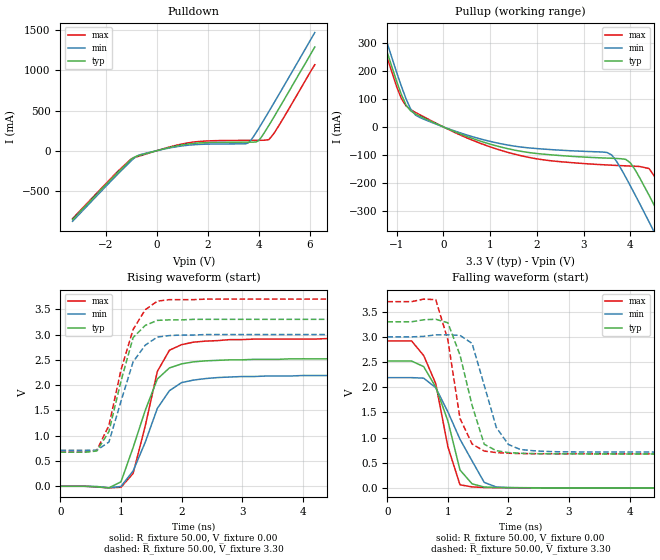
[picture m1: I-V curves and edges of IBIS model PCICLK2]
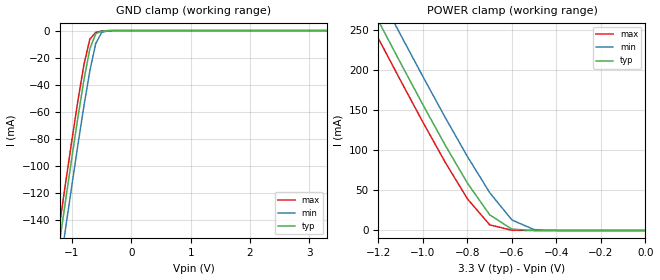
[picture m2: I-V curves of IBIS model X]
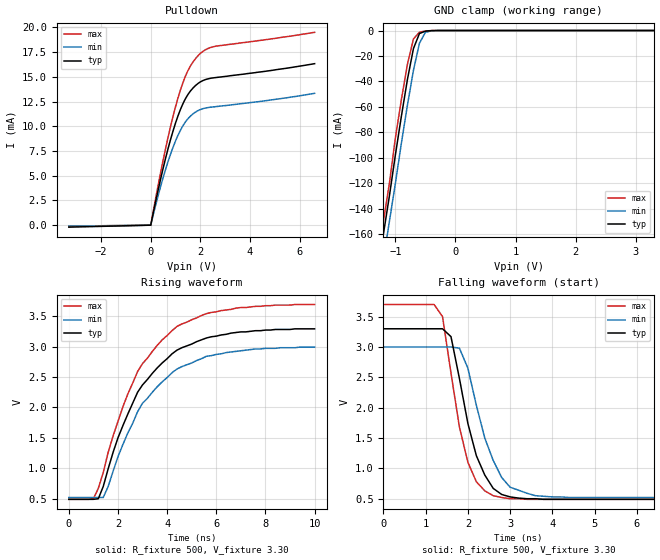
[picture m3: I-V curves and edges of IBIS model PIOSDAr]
|   * 9250-28.ibs * IBIS 2.1 Model for ICS9250-28
| Rev History
| Rev No.   Description
| 1.0   Initial release with Updated Parasitic Parameters
[IBIS Ver]   2.1
[Comment char]  |_char
[File name]   9250-28.ibs
[Date]   Aug 15, 2002
[File Rev]   1.1
[Source]   Originated at Integrated Circuit Systems, Inc.
[Disclaimer]
(C) Copyright Integrated Circuit Systems, Inc. 1997
   All rights reserved
ICS hereby grants the user of this IBIS model a non-exclusive,
nontransferable license to use this IBIS model under the following terms.
Before using this IBIS model, the user should read this license.
If the user does not accept these terms,  the IBIS model should be
returned to ICS within 30 days.
   The user is granted this license only to use the IBIS model and
is not granted rights to sell, load, rent, lease or license the IBIS
model in whole or in part, or in modified form to anyone other than
user. User may modify the IBIS model to suit its specific
applications but rights to derivative works and such modifications
shall belong to ICS.
   This IBIS model is provided on an "AS IS" basis and ICS makes
absolutely no warranty with respect to the information contained
herein. ICS DISCLAIMS AND CUSTOMER WAIVES ALL WARRANTIES, EXPRESS
OR IMPLIED, INCLUDING WARRANTIES OF MERCHANTABILITY OR FITNESS FOR
A PARTICULAR PURPOSE. The entire risk as to quality and performance
is with the Customer. ACCORDINGLY, IN NO EVENT SHALL THE COMPANY BE
LIABLE FOR ANY DAMAGES, WHETHER IN CONTRACT OR TORT,INCLUDING ANY
LOST PROFITS OR OTHER INCIDENTAL, CONSEQUENTIAL, EXEMPLARY, OR
PUNITIVE DAMAGES ARISING OUT OF THE USE OR APPLICATION OF THE IBIS
model provided in this package. Further, ICS reserves the right to
make changes without notice to any product herein to improve
reliability, function, or design. ICS does not convey any license
under patent rights or any other intellectual property rights,
including those of third parties.
   ICS is not obligated to provide maintenance or support
for the licensed IBIS model.
|   COMPONENT: ICS9250-28
[Component]   ICS9250-28
[Manufacturer]  ICS
[Package]
| variable   typ   min   max
R_pkg   81.1m   62.2m   100.0m
L_pkg   6.7nH   4.9nH   8.5nH
C_pkg   0.53pF  0.21pF  0.85pF
[Pin]   signal_name   model_name   R_pin   L_pin   C_pin
1   IOAPIC   IOAPIC
2   VDDL   POWER
3   GNDL   GND
4   FS2/REF0   PIO17
5   VDD   POWER
6   X1   X
7   X2   X
8   GND   GND
9   VDD   POWER
10   3V66-0   3V661
11   3V66-1   3V661
12   3V66-2   3V661
13   GND   GND
14   VDD   POWER
15   PCICLK0   PCICLK2
16   PCICLK1   PCICLK2
17   GND   GND
18   FS0   FS
19   GND   GND
20   VDD   POWER
21   PD#   PD
22   SCLK   SCLK
23   SDATA   PIOSDAr
24   GND   GND
25   VDD   POWER
26   48MHz_0   48MH
27   48MHz_1   48MHz2
28   FS1   FS
29   SDRAM12   SDRAM5
30   GND   GND
31   VDD   POWER
32   SDRAM11   SDRAM5
33   SDRAM10   SDRAM5
34   GND   GND
35   VDD   POWER
36   SDRAM9   SDRAM5
37   SDRAM8   SDRAM5
38   SDRAM7   SDRAM5
39   GND   GND
40   VDD   POWER
41   SDRAM6   SDRAM5
42   SDRAM5   SDRAM5
43   GND   GND
44   VDD   POWER
45   SDRAM4   SDRAM5
46   SDRAM3   SDRAM5
47   SDRAM2   SDRAM5
48   GND   GND
49   VDD   POWER
50   SDRAM1   SDRAM5
51   SDRAM0   SDRAM5
52   GND   GND
53   CPUCLK1   CPU5
54   CPUCLK0   CPU5
55   GNDL   GND
56   VDDL   POWER
| Models and submodels in the file (13): PCICLK2 (Output), 3V661 (Output), X (Input), PIOSDAr (I/O_open_drain), SCLK (Input), FS (Input), PD (Input), 48MHz2 (Output), 48MH (Output), SDRAM5 (Output), IOAPIC (Output), CPU5 (Output), PIO17 (I/O)
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|*  Either 3.3V or 2.5V
|** All model are simulated with typical corner process
|   Model PCICLK2
[Model]   PCICLK2
Model_type   Output
Polarity   Non-Inverting
Vmeas = 1.5V
Cref = 30pF
Rref = 0
Vref = 1.5V
C_comp   5.50pF   5.00pF   6.00pF
[Temperature Range]   27.00   70.00   0.00
[Voltage Range]   3.30V   3.00V   3.70V
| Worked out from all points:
|   slope of the pulldown table from 0 to 0.495 V, typ, clamps not added: 12.4 ohm
|   slope of the pullup table from 0 to 0.495 V, typ, clamps not added: 14.7 ohm
|   rising waveform, R_fixture 50.00, V_fixture 0.00: 20-80 % time 444ps typ, 474ps min, 361ps max; typ from 0 V to 2.52 V
|   rising waveform, R_fixture 50.00, V_fixture 3.30: 20-80 % time 338ps typ, 377ps min, 384ps max; typ from 0.674 V to 3.3 V
|   falling waveform, R_fixture 50.00, V_fixture 0.00: 20-80 % time 377ps typ, 546ps min, 357ps max; typ from 2.52 V to 0 V
|   falling waveform, R_fixture 50.00, V_fixture 3.30: 20-80 % time 356ps typ, 339ps min, 278ps max; typ from 3.3 V to 0.674 V
[Pulldown]
| voltage   I(typ)   I(min)   I(max)
-3.3V     -857.9mA   -878.4mA   -845.3mA
-1.5V     -261.3mA   -282.1mA   -248.7mA
-1V       -107.9mA   -125mA     -102.2mA
-700mV    -61.18mA   -54.61mA   -68.48mA
400mV     32.81mA    27.49mA    37.39mA
1.3V      86.08mA    70.47mA    101mA
3.6V      106.5mA    98.57mA    128.8mA
3.9V      108.8mA    225.9mA    129.5mA
4V        126.6mA    276.5mA    129.7mA
4.4V      314.9mA    487.2mA    137.4mA
4.8V      527.7mA    703mA      316.3mA
6.2V      1.29A      1.47A      1.07A
[Pullup]
| voltage   I(typ)   I(min)   I(max)
-3.3V     1.4A       1.43A      1.38A
-1.5V     421.2mA    455.2mA    400.3mA
-900mV    116.5mA    146.2mA    102mA
-700mV    57.52mA    63.85mA    61.81mA
-500mV    38.48mA    33.44mA    43.28mA
1.4V      -78.79mA   -65.56mA   -92.19mA
3.5V      -111.7mA   -91.56mA   -136.3mA
4V        -128.7mA   -211.2mA   -140.2mA
4.4V      -245.1mA   -340.5mA   -149.2mA
4.8V      -375.8mA   -472.8mA   -260.1mA
5.2V      -509mA     -606.4mA   -391.1mA
6.2V      -845.7mA   -943.1mA   -726.8mA
[Ramp]
| variable   typ   min   max
dV/dt_r   1.51/354.04p   1.31/416.22p   1.75/312.34p
dV/dt_f   1.58/300.00p   1.37/300.00p   1.81/300.00p
[Rising Waveform]
R_fixture = 50.00
V_fixture = 0.00
V_fixture_min = 0.00
V_fixture_max = 0.00
| time   V(typ)   V(min)   V(max)
0s        0V         0V         0V
800ps     -31.01mV   -29.88mV   -31.17mV
1ns       89.14mV    -3.03mV    -19.9mV
1.2ns     765.6mV    303mV      254mV
1.4ns     1.5V       870.1mV    1.19V
1.6ns     2.12V      1.54V      2.27V
1.8ns     2.34V      1.89V      2.69V
2ns       2.42V      2.05V      2.8V
3.4ns     2.51V      2.18V      2.91V
10ns      2.52V      2.19V      2.92V
[Rising Waveform]
R_fixture = 50.00
V_fixture = 3.30
V_fixture_min = 3.00
V_fixture_max = 3.70
| time   V(typ)   V(min)   V(max)
0s        673.6mV    711.3mV    675.9mV
400ps     673.6mV    711.3mV    675.9mV
600ps     696.8mV    712.9mV    712.6mV
800ps     1.08V      874mV      1.2V
1ns       2.08V      1.68V      2.3V
1.2ns     2.94V      2.46V      3.1V
1.4ns     3.18V      2.79V      3.49V
1.6ns     3.28V      2.95V      3.66V
2.4ns     3.3V       3V         3.7V
10ns      3.3V       3V         3.7V
[Falling Waveform]
R_fixture = 50.00
V_fixture = 0.00
V_fixture_min = 0.00
V_fixture_max = 0.00
| time   V(typ)   V(min)   V(max)
0s        2.52V      2.19V      2.92V
400ps     2.52V      2.19V      2.92V
600ps     2.41V      2.18V      2.63V
800ps     2V         1.99V      2.07V
1ns       1.33V      1.51V      817.2mV
1.2ns     355.4mV    965.6mV    60.84mV
1.4ns     79.4mV     534.8mV    19.11mV
1.6ns     15.91mV    109mV      7.22mV
1.8ns     6.17mV     16.27mV    3.69mV
10ns      0V         1.56uV     652.7nV
[Falling Waveform]
R_fixture = 50.00
V_fixture = 3.30
V_fixture_min = 3.00
V_fixture_max = 3.70
| time   V(typ)   V(min)   V(max)
0s        3.3V       3V         3.7V
800ps     3.35V      3.04V      3.74V
1ns       3.28V      3.04V      2.94V
1.2ns     2.64V      3.03V      1.38V
1.4ns     1.64V      2.87V      871.5mV
1.6ns     866.9mV    2.04V      731.3mV
1.8ns     737.7mV    1.2V       700.7mV
2ns       701.1mV    861.1mV    687.7mV
2.2ns     687.2mV    761.6mV    681.9mV
10ns      673.6mV    711.3mV    675.9mV
|   Model X
[Model]   X
Model_type   Input
Polarity   Non-Inverting
Vinl = 800.00mV
Vinh =   2.00V
C_comp   5.50pF   5.00pF   6.00pF
[Temperature Range]   27.00   70.00   0.00
[Voltage Range]   3.30V   3.00V   3.70V
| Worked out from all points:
|   GND clamp passes 1 mA (typ) near -0.53 V on its own axis
|   POWER clamp passes 1 mA (typ) near -0.56 V on its own axis
[GND_clamp]
| voltage   I(typ)   I(min)   I(max)
-3.3V     -818.7mA   -838.4mA   -806.5mA
-1.3V     -184.4mA   -205.1mA   -171.6mA
-1.2V     -153.6mA   -174.3mA   -140.8mA
-1.1V     -123.2mA   -143.8mA   -110.3mA
-1V       -93.23mA   -113.8mA   -80.48mA
-900mV    -64.14mA   -84.35mA   -51.7mA
-800mV    -36.72mA   -56.02mA   -25.33mA
-700mV    -13.63mA   -29.93mA   -6.41mA
-600mV    -2.31mA    -9.53mA    -1.31mA
-500mV    -487.9uA   -1.36mA    -326.3uA
-400mV    -91uA      -228.6uA   -44.4uA
3.3V      108.9pA    1.5uA      48.42pA
[POWER_clamp]
| voltage   I(typ)   I(min)   I(max)
-3.3V     1.41A      1.44A      1.39A
-1.3V     314.3mA    349.5mA    292.4mA
-1.2V     261.1mA    296.3mA    239.1mA
-1.1V     208.4mA    243.6mA    186.5mA
-1V       156.6mA    191.7mA    134.8mA
-900mV    106.3mA    140.8mA    85.01mA
-800mV    58.94mA    92.02mA    39.34mA
-700mV    19.46mA    47.14mA    7mA
-600mV    1.61mA     13.03mA    241.9uA
-500mV    48.08uA    1.03mA     4.48uA
-400mV    1.09uA     42.41uA    71.42nA
0V        108.9pA    1.22nA     66.46pA
|   Model PIOSDAr
[Model]   PIOSDAr
Model_type   I/O_open_drain
Polarity   Inverting
Enable   Active-High
Vinl =   0.80V
Vinh =   2.00V
C_comp   5.50pF   5.00pF   6.00pF
[Temperature Range]   27.00   70.00   0.000
[Voltage Range]   3.30V   3.00V   3.70V
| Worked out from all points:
|   slope of the pulldown table from 0 to 0.495 V, typ, clamps not added: 86.7 ohm
|   GND clamp passes 1 mA (typ) near -0.53 V on its own axis
|   rising waveform, R_fixture 500, V_fixture 3.30: 20-80 % time 2.16ns typ, 2.16ns min, 2.15ns max; typ from 0.49 V to 3.29 V
|   falling waveform, R_fixture 500, V_fixture 3.30: 20-80 % time 574ps typ, 634ps min, 494ps max; typ from 3.3 V to 0.49 V
[Pulldown]
| voltage   I(typ)   I(min)   I(max)
-3.3V     -200uA     -100uA     -100uA
0V        0A         0A         -12.81pA
300mV     3.57mA     3mA        4.06mA
600mV     6.79mA     5.66mA     7.77mA
900mV     9.54mA     7.89mA     11.03mA
1.1V      11.07mA    9.11mA     12.88mA
1.3V      12.3mA     10.07mA    14.43mA
1.5V      13.22mA    10.77mA    15.64mA
1.8V      14.11mA    11.43mA    16.83mA
2.1V      14.62mA    11.78mA    17.57mA
2.6V      14.92mA    11.98mA    18.09mA
6.6V      16.33mA    13.33mA    19.5mA
[GND_clamp]
| voltage   I(typ)   I(min)   I(max)
-3.3V     -860mA     -880mA     -840mA
-1.3V     -190mA     -210mA     -180mA
-1.2V     -160mA     -180mA     -150mA
-1.1V     -130mA     -150mA     -120mA
-1V       -97.6mA    -120mA     -84.25mA
-900mV    -67.14mA   -88.3mA    -54.11mA
-800mV    -38.43mA   -58.65mA   -26.49mA
-700mV    -14.23mA   -31.32mA   -6.64mA
-600mV    -2.36mA    -9.93mA    -1.32mA
-500mV    -490uA     -1.38mA    -330uA
-400mV    -91.06uA   -230uA     -44.42uA
3.3V      110pA      1.56nA     57.23pA
[Ramp]
| variable   typ   min   max
dV/dt_r   1.68/2.17n   1.48/2.18n   1.92/2.16n
dV/dt_f   1.69/0.55n   1.49/0.63n   1.93/0.48n
R_load = 500
[Rising Waveform]
R_fixture = 500
V_fixture = 3.30
V_fixture_min = 3.00
V_fixture_max = 3.70
| time   V(typ)   V(min)   V(max)
0s        490mV      520mV      490mV
1ns       490mV      520mV      500mV
1.2ns     500mV      520mV      670mV
1.4ns     700mV      520mV      930mV
2ns       1.5V       1.19V      1.77V
2.8ns     2.25V      1.93V      2.59V
4.4ns     2.94V      2.63V      3.33V
5.6ns     3.14V      2.84V      3.54V
6.8ns     3.23V      2.92V      3.63V
10ns      3.29V      2.99V      3.69V
[Falling Waveform]
R_fixture = 500
V_fixture = 3.30
V_fixture_min = 3.00
V_fixture_max = 3.70
| time   V(typ)   V(min)   V(max)
0s        3.3V       3V         3.7V
1.2ns     3.3V       3V         3.7V
1.4ns     3.3V       3V         3.5V
1.6ns     3.17V      3V         2.57V
2ns       1.74V      2.65V      1.1V
2.2ns     1.21V      2.04V      780mV
2.6ns     670mV      1.13V      550mV
3ns       530mV      690mV      500mV
3.6ns     500mV      550mV      490mV
10ns      490mV      520mV      490mV
